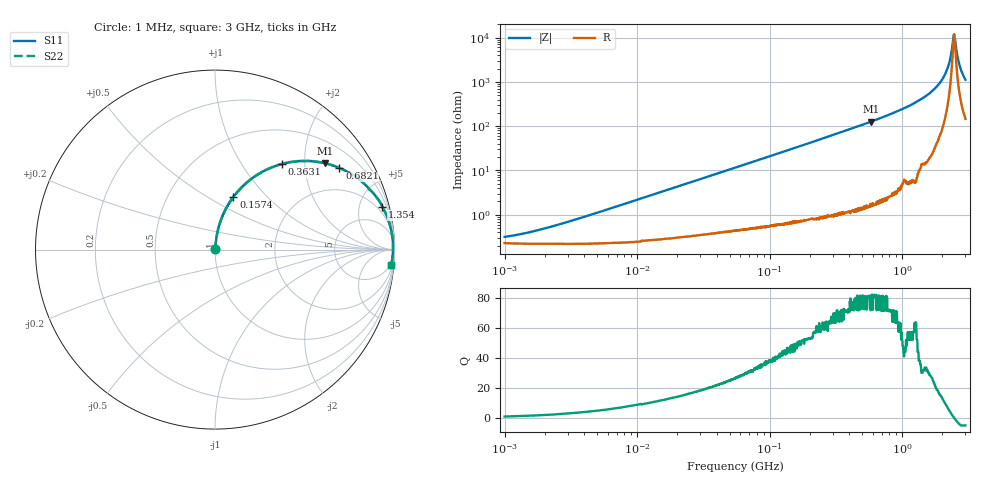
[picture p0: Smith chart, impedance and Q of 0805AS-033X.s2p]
!s-Parameter Generated by FASTRON Sdn. Bhd.
!FASTRON P/N : 0805AS-033X
!Keysight Technologies: E4991B_MY54100416_A.01.15
!Date: Mon Jun 15 12:50:06 2026
!Version  :Rev01  Mon Jun 15 12:50:06 2026
!Data & Calibration Information:
!Freq  S11  S21  S12  S22
!PortZ  Port1:50+j0  Port2:50+j0
!When reading reference impedance value at option line is always used.
! Remarks : This data is being provided solely for informational purposes.
# Hz S dB R 50
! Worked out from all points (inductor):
!   1601 points, 1 MHz to 3 GHz, reference 50 ohm
!   read as one part in series: L = 34.7 nH near 3.022 MHz
!   highest Q = 81.4 at 581.2 MHz (marker M1), where L = 34.6 nH
!   self-resonance near 2.456 GHz
!   S11 on the Smith chart (normalised r, x): 1 MHz: 1.00, +0.00; 157.4 MHz: 1.01, +0.65; 363.1 MHz: 1.02, +1.53; 682.1 MHz: 1.04, +3.03; 1.354 GHz: 1.20, +7.79; 3 GHz: 4, -22
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1000000  -50.00 43.6  -0.02 -0.1  -0.02 -0.1  -50.00 43.6
1649378  -47.50 58.2  -0.02 -0.2  -0.02 -0.2  -47.50 58.2
3804036  -41.40 74.7  -0.02 -0.5  -0.02 -0.5  -41.40 74.7
1.447069e7  -30.10 83.2  -0.03 -1.8  -0.03 -1.8  -30.10 83.2
5.504702e7  -18.80 81.3  -0.10 -6.6  -0.10 -6.6  -18.80 81.3
1.574367e8  -10.20 70.7  -0.50 -18.1  -0.50 -18.1  -10.20 70.7
2.083556e8  -8.04 65.6  -0.81 -23.3  -0.81 -23.3  -8.04 65.6
3.631036e8  -4.38 52.1  -2.06 -37.1  -2.06 -37.1  -4.38 52.1
5.81181e8  -2.17 38.1  -4.20 -51.2  -4.20 -51.2  -2.17 38.1
6.821091e8  -1.63 33.2  -5.22 -56.0  -5.22 -56.0  -1.63 33.2
7.925923e8  -1.21 28.8  -6.35 -60.4  -6.35 -60.4  -1.21 28.8
1.353887e9  -0.33 14.3  -12.20 -74.2  -12.20 -74.2  -0.33 14.3
1.712864e9  -0.15 8.7  -16.40 -79.0  -16.40 -79.0  -0.15 8.7
2.03054e9  -0.09 4.7  -21.70 -80.7  -21.70 -80.7  -0.09 4.7
2.23307e9  -0.07 2.4  -27.40 -78.0  -27.40 -78.0  -0.07 2.4
2.301132e9  -0.07 1.7  -30.30 -74.3  -30.30 -74.3  -0.07 1.7
2.39512e9  -0.07 0.7  -36.60 -57.2  -36.60 -57.2  -0.07 0.7
2.455801e9  -0.07 0.1  -41.40 -13.7  -41.40 -13.7  -0.07 0.1
2.530652e9  -0.08 -0.6  -37.30 50.5  -37.30 50.5  -0.08 -0.6
2.647227e9  -0.08 -1.7  -30.00 71.5  -30.00 71.5  -0.08 -1.7
2.75535e9  -0.10 -2.8  -26.20 75.7  -26.20 75.7  -0.10 -2.8
3e9  -0.13 -5.0  -21.10 77.5  -21.10 77.5  -0.13 -5.0
